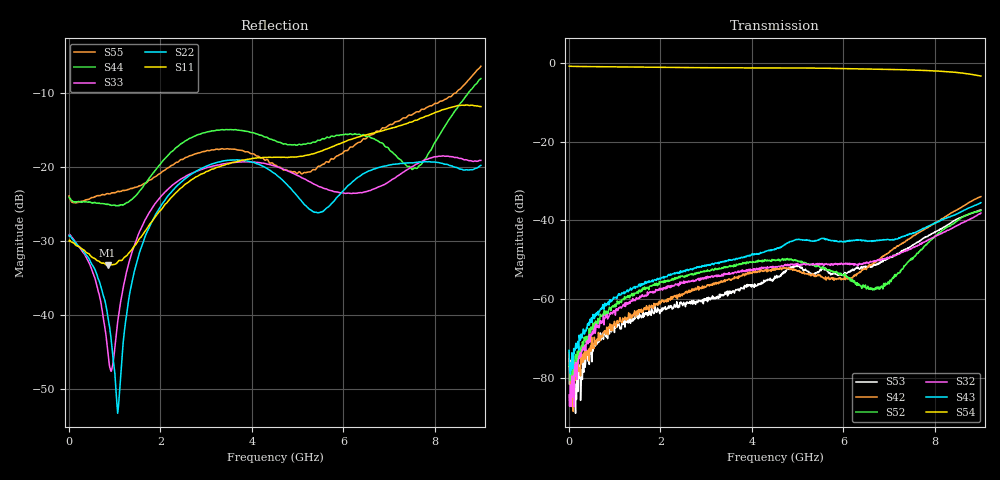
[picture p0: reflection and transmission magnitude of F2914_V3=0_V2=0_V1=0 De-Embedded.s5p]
! Integrated Device Technology
! Corporate Headquarters
! 6024 Silver Creek Valley Road
! San Jose, CA 95138  USA
! Phone:  1-408-284-8200
! Toll Free:  1-800-223-1366
! Webpage:  http://www.idt.com/
! Timing and RF Division
! 515 Groton Road, Suite 102
! Westford, MA 01886-6024
! Device:  F2914
! Description: High Reliability SP4T RF Switch
! Frequency:  0.05 -  8.GHz
! Package:  4x4 mm Thin QFN Plastic Package: 24 pin
! Ports:  5 RF,  5 DC
!  Pin  1  = GND
!  Pin  2  = GND
!  Pin  3  = GND
!  Pin  4  = GND
!  Pin  5  = RF4  =  Port 4
!  Pin  6  = GND
!  Pin  7  = GND
!  Pin  8  = RF3  =  Port 3
!  Pin  9  = GND
!  Pin 10  = GND
!  Pin 11  = RF2  =  Port 2
!  Pin 12  = GND
!  Pin 13  = GND
!  Pin 14  = RF1  =  Port 1
!  Pin 15  = GND
!  Pin 16  = Vcc
!  Pin 17  = V1
!  Pin 18  = V2
!  Pin 19  = V3
!  Pin 20  = VSSext
!  Pin 21  = GND
!  Pin 22  = RFC  =  Port 5
!  Pin 23  = GND
!  Pin 24  = GND
! Voltage:  VDD  =  +3.30 Volts
!  VSSEXT =  0.00 Volts
! Current:  IDD  = 317  uA
! State:  RF1 Selected
! V1:  Logic LOW
! V2:  Logic LOW
! V3:  Logic LOW
! Data:  The device was measured on the F291x evaluation board which has
!  individual transmission lines to the RF pins.  Data was collected
!  using a calibrated network analyzer.  The input lines were
!  modeled using Automatic Fixture Removal (AFR) from Keysight.
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# Hz S  dB  R 50
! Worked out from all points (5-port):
!   900 points, 10 MHz to 9 GHz, reference 50 ohm
!   strongest paths, dB at 10 MHz, 2.26 GHz, 4.51 GHz, 6.76 GHz, 9 GHz:
!     S54: -0.8, -1.1, -1.2, -1.5, -3.3
!     S43: -73.0, -53.7, -47.4, -45.1, -35.5
!     S32: -84.4, -56.7, -51.9, -50.0, -38.1
!     S52: -77.0, -54.8, -50.2, -57.5, -37.5
!     S42: -73.6, -60.0, -52.1, -50.2, -33.9
!     S53: -74.9, -62.6, -54.6, -50.9, -37.3
!   lowest |S11| = -33.3 dB at 850 MHz (marker M1), VSWR 1.04, Z = 48.6 + j1.59 ohm
!   |S11| at or under -10 dB: start of sweep to end of sweep
